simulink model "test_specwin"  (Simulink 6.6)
settings: Solver=ode45  StartTime=0.0  StopTime=10.0  RelTol=1e-3
libraries: sltpda x2

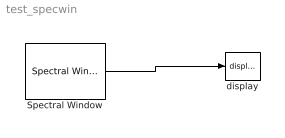
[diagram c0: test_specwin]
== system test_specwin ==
  Spectral Window : sltpda/AO class/Spectral Window  SystemSampleTime=-1  wname=Hanning  wlen=100  psll=0
  display : sltpda/AO class/display  Tag=display  SystemSampleTime=-1
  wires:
  Spectral Window/1 -> display/1
